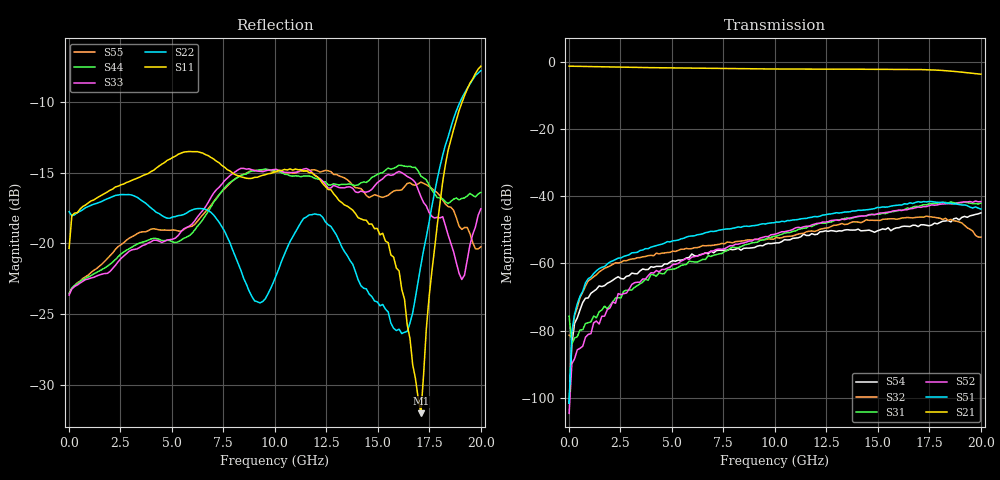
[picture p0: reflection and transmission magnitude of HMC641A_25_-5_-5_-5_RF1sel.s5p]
! Device:  HMC641A
! Description: GaAs MMIC SP4T NON-REFLECTIVE
! Frequency:  0.01 -  18 GHz
! Ports:
! RFC = Port 1
! RF1 = Port 2
! RF2 = Port 3
! RF3 = Port 4
! RF4 = Port 5
! State: RF1 selected
! Vss:  -5 Volts
! Control A  -5 Volts
! Control B:  -5 Volts
! Temperature = +25 C
! Data: Data was collected using a calibrated network analyzer.
!  The reference plane is the edge of the device.
! Note: Analog Devices supplies this data as a sample of measured data for this product.
!  Your particular data for this product may vary.
!  Analog Devices reserves the right to change this data at anytime
# Hz S DB R 50.0
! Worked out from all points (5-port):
!   152 points, 10 MHz to 20.01 GHz, reference 50 ohm
!   strongest paths, dB at 10 MHz, 5.043 GHz, 10.08 GHz, 15.11 GHz, 20.01 GHz:
!     S21: -1.2, -1.7, -2.0, -2.1, -3.6
!     S51: -101.6, -53.3, -47.6, -43.3, -43.8
!     S52: -104.7, -60.3, -51.2, -44.9, -41.5
!     S31: -75.7, -61.7, -51.9, -45.3, -42.0
!     S32: -81.4, -56.3, -52.2, -47.2, -52.2
!     S54: -101.7, -59.2, -53.9, -50.0, -44.9
!   lowest |S11| = -32.0 dB at 17.1 GHz (marker M1), VSWR 1.05, Z = 52.5 + j0.502 ohm
!   |S11| at or under -10 dB: start of sweep to 19.1 GHz
